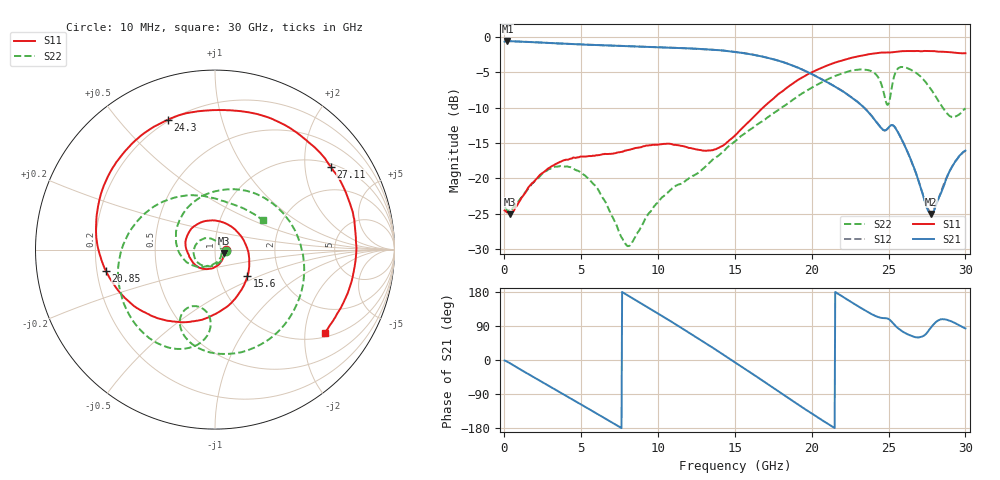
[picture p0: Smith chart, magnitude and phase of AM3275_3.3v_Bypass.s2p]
!Keysight Technologies,N5245B,MY58422270,A.16.20.02
!Date: Monday, May 05, 2025 22:34:11
!Correction: S11(C  2-Port  )
!S21(C  2-Port  )
!S12(C  2-Port  )
!S22(C  2-Port  )
!S2P File: Measurements: S11, S21, S12, S22:
# Hz S  dB  R 50
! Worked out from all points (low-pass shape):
!   801 points, 10 MHz to 30 GHz, reference 50 ohm
!   highest |S21| = -0.57 dB at 197.4 MHz (marker M1); lowest = -25.0 dB at 27.75 GHz (marker M2)
!   |S21| within 3 dB of the highest: start of sweep to 18.16 GHz
!   lowest |S11| = -25.1 dB at 347.4 MHz (marker M3), VSWR 1.12, Z = 55.4 - j2.35 ohm
!   |S11| at or under -10 dB: start of sweep to 16.82 GHz
!   |S22| runs from -29.6 to -4.2 dB; largest |S21 - S12| = 0.018
!   S11 on the Smith chart (normalised r, x): 10 MHz: 1.13, -0.01; 15.6 GHz: 1.36, -0.43; 20.85 GHz: 0.24, -0.09; 24.3 GHz: 0.19, +0.69; 27.11 GHz: 1.09, +2.72; 30 GHz: 1.12, -2.53
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1e7  -24.54 -2.6  -0.66 -1.4  -0.49 -1.5  -24.05 -8.8
1.974375e8  -24.81 -13.6  -0.57 -4.8  -0.56 -4.9  -24.65 -13.7
3.473875e8  -25.06 -22.3  -0.59 -8.4  -0.60 -8.5  -24.57 -23.3
2.784075e9  -18.69 -110.3  -0.84 -66.1  -0.82 -66.0  -18.88 -130.6
5.033325e9  -16.91 -149.2  -1.06 -118.5  -1.06 -118.6  -19.24 163.4
7.582475e9  -16.26 -174.6  -1.27 -178.8  -1.26 -178.9  -28.23 59.6
8.182275e9  -15.95 179.1  -1.31 166.7  -1.30 166.7  -29.44 11.5
1.001916e10  -15.23 150.6  -1.46 121.9  -1.45 121.9  -23.25 -79.0
1.226841e10  -15.78 91.3  -1.64 65.6  -1.65 65.6  -19.61 -117.2
1.373042e10  -15.87 33.3  -1.84 27.8  -1.83 27.7  -17.08 -137.5
1.5005e10  -13.94 -18.4  -2.11 -6.0  -2.11 -6.0  -14.76 -163.5
1.56048e10  -12.61 -39.4  -2.29 -22.2  -2.28 -22.2  -13.72 -179.8
1.77041e10  -8.31 -96.8  -3.26 -79.2  -3.28 -79.4  -10.50 108.3
2.002832e10  -4.97 -150.1  -5.28 -142.1  -5.27 -142.1  -7.15 23.1
2.085305e10  -4.16 -168.8  -6.22 -163.4  -6.21 -163.4  -6.17 -3.5
2.298984e10  -2.75 142.1  -9.20 142.5  -9.19 142.2  -4.62 -65.8
2.43019e10  -2.27 109.8  -12.28 113.6  -12.30 113.3  -5.63 -107.4
2.501416e10  -2.19 91.3  -12.78 107.9  -12.77 107.9  -9.35 -100.0
2.568894e10  -2.05 74.2  -13.80 81.6  -13.77 81.5  -4.34 -117.2
2.711346e10  -2.01 35.7  -21.45 61.2  -21.47 60.1  -5.66 -179.7
2.775075e10  -1.99 18.5  -25.02 84.8  -24.79 84.3  -7.37 148.9
3e10  -2.30 -37.3  -16.07 83.3  -16.10 83.0  -10.09 31.7
